| IBIS file ussst2gxxac.ibs created by s2ibis3 verion 1.1
| North Carolina State University, ERL, 2006
| This Model is valid for Commercial Temperature Range 0C<=Tc<=95C
| Valid for DDR2-400/533/667/800/1067 operation
| Part Number   VDD/VDDQ   Package   Architecture
| SCB18T2G160AF   1.8 +0.1/-0.1   84-Ball FBGA   128Meg x 16
| SCB18T2G800AF   1.8 +0.1/-0.1   60-Ball FBGA   256Meg x 8
| SCN18T2G160AF   1.8 +0.1/-0.1   84-Ball FBGA   128Meg x 16
| SCN18T2G800AF   1.8 +0.1/-0.1   60-Ball FBGA   256Meg x 8
| TOPR: Operating Temperature
[IBIS Ver]   3.2
[File name]  ussst2gxxac.ibs
[File Rev]   1.6
[Date]   2016-09-17
[Source]   Simulation of a silicon level SPICE model
[Notes]   IBIS Characteristics for I/O Buffer
   IBIS Model Revision History:
Rev 1.3: 2014-10-14
   - IBIS model file initial creation
Rev 1.3: 2016-09-01
   - update model ODT_75 and ODT_150;
Rev 1.3: 2016-09-05
   - update x16 UDQS#/UDQS/UDM/LDQS#/LDQS/LDM model information;
   - update x8  RDQS#/DM_RDQS model information;
   - add new model RDQS;
Rev 1.4: 2016-09-05
   - correct support speed
   - change RDQS#/DM_RDQS model style
Rev 1.5: 2016-09-08
   - update data to support DDR2-800/1067
Rev 1.6: 2016-09-17
   - split and update "DATA_FULL_800" & "DATA_REDUCED_800"
   and  "DATA_FULL_1067" & "DATA_REDUCED_1067"
   "rising" & "falling" wave data;
   - update ODT "power clamp" data to touch zero current point.
[disclaimer] The IBIS models are for modeling purpose only and are
   subject to change without any notice. UniIC is not
   responsible for any problems the models may cause.
[Copyright]  Copyright 2016 UniIC Semiconductors Corp. All rights reserved
|   Component: SCB18T2G160AF
[Component]   SCB18T2G160AF
[Manufacturer]   UniIC Semiconductors Corp.
| All balls excluding NC, POWER and GND (R[Ohm], L[H], C[F])
[Package]   | FBGA-84 Ball
|Variable   typ   min   max
R_pkg   3.54E-01   2.15E-01   4.22E-01
L_pkg   1.74E-09   9.52E-10   2.26E-09
C_pkg   5.49E-13   3.07E-13   7.49E-13
[Pin]   signal_name model_name   R_pin   L_pin   C_pin
A1   VDD   POWER   NA   NA   NA
A3   VSS   GND   NA   NA   NA
A7   VSSQ   GND   NA   NA   NA
A8   UDQS#   DQ   3.91E-01   1.89E-09   6.31E-13
A9   VDDQ   POWER   NA   NA   NA
B1   DQ14   DQ   3.94E-01   1.93E-09   6.78E-13
B2   VSSQ   GND   NA   NA   NA
B3   UDM   DM   4.00E-01   1.72E-09   6.23E-13
B7   UDQS   DQ   3.85E-01   1.79E-09   6.17E-13
B8   VSSQ   GND   NA   NA   NA
B9   DQ15   DQ   4.04E-01   1.94E-09   6.87E-13
C1   VDDQ   POWER   NA   NA   NA
C2   DQ9   DQ   3.30E-01   1.58E-09   6.19E-13
C3   VDDQ   POWER   NA   NA   NA
C7   VDDQ   POWER   NA   NA   NA
C8   DQ8   DQ   3.86E-01   1.81E-09   6.25E-13
C9   VDDQ   POWER   NA   NA   NA
D1   DQ12   DQ   4.15E-01   2.16E-09   7.19E-13
D2   VSSQ   GND   NA   NA   NA
D3   DQ11   DQ   3.58E-01   1.84E-09   4.33E-13
D7   DQ10   DQ   3.59E-01   1.54E-09   6.33E-13
D8   VSSQ   GND   NA   NA   NA
D9   DQ13   DQ   3.88E-01   1.80E-09   6.09E-13
E1   VDD   POWER   NA   NA   NA
E3   VSS   GND   NA   NA   NA
E7   VSSQ   GND   NA   NA   NA
E8   LDQS#   DQ   3.29E-01   1.47E-09   5.27E-13
E9   VDDQ   POWER   NA   NA   NA
F1   DQ6   DQ   3.57E-01   1.72E-09   6.81E-13
F2   VSSQ   GND   NA   NA   NA
F3   LDM   DM   3.66E-01   1.80E-09   4.94E-13
F7   LDQS   DQ   3.51E-01   1.65E-09   4.51E-13
F8   VSSQ   GND   NA   NA   NA
F9   DQ7   DQ   3.45E-01   1.65E-09   5.83E-13
G1   VDDQ   POWER   NA   NA   NA
G2   DQ1   DQ   3.74E-01   1.80E-09   5.29E-13
G3   VDDQ   POWER   NA   NA   NA
G7   VDDQ   POWER   NA   NA   NA
G8   DQ0   DQ   3.89E-01   1.76E-09   7.05E-13
G9   VDDQ   POWER   NA   NA   NA
H1   DQ4   DQ   4.00E-01   1.95E-09   6.62E-13
H2   VSSQ   GND   NA   NA   NA
H3   DQ3   DQ   3.99E-01   1.92E-09   4.51E-13
H7   DQ2   DQ   3.73E-01   1.57E-09   6.01E-13
H8   VSSQ   GND   NA   NA   NA
H9   DQ5   DQ   3.76E-01   1.57E-09   6.31E-13
J1   VDDL   POWER   NA   NA   NA
J2   VREF   POWER   NA   NA   NA
J3   VSS   GND   NA   NA   NA
J7   VSSDL   GND   NA   NA   NA
J8   CK   CLKCA_RCV   2.92E-01   1.50E-09   4.65E-13
J9   VDD   POWER   NA   NA   NA
K2   CKE   CLKCA_RCV   2.87E-01   1.53E-09   4.36E-13
K3   WE#   CLKCA_RCV   2.26E-01   1.11E-09   3.27E-13
K7   RAS#   CLKCA_RCV   2.27E-01   9.78E-10   3.41E-13
K8   CK#   CLKCA_RCV   2.98E-01   1.41E-09   5.62E-13
K9   ODT   CLKCA_RCV   3.79E-01   1.97E-09   7.49E-13
L1   BA2   CLKCA_RCV   3.69E-01   2.26E-09   5.19E-13
L2   BA0   CLKCA_RCV   3.48E-01   1.83E-09   4.55E-13
L3   BA1   CLKCA_RCV   2.17E-01   9.61E-10   3.07E-13
L7   CAS#   CLKCA_RCV   2.15E-01   9.52E-10   4.00E-13
L8   CS#   CLKCA_RCV   2.95E-01   1.43E-09   5.20E-13
M2   A10   CLKCA_RCV   3.56E-01   1.93E-09   5.14E-13
M3   A1   CLKCA_RCV   3.41E-01   1.90E-09   3.68E-13
M7   A2   CLKCA_RCV   3.40E-01   1.79E-09   4.49E-13
M8   A0   CLKCA_RCV   3.54E-01   1.82E-09   5.67E-13
M9   VDD   POWER   NA   NA   NA
N1   VSS   GND   NA   NA   NA
N2   A3   CLKCA_RCV   3.46E-01   1.82E-09   5.59E-13
N3   A5   CLKCA_RCV   3.56E-01   1.85E-09   5.59E-13
N7   A6   CLKCA_RCV   3.76E-01   1.76E-09   6.49E-13
N8   A4   CLKCA_RCV   3.52E-01   1.90E-09   4.89E-13
P2   A7   CLKCA_RCV   3.86E-01   1.97E-09   6.01E-13
P3   A9   CLKCA_RCV   4.08E-01   2.11E-09   4.37E-13
P7   A11   CLKCA_RCV   4.01E-01   2.17E-09   5.49E-13
P8   A8   CLKCA_RCV   3.87E-01   1.85E-09   5.76E-13
P9   VSS   GND   NA   NA   NA
R1   VDD   POWER   NA   NA   NA
R2   A12   CLKCA_RCV   4.22E-01   2.07E-09   6.47E-13
R8   A13   CLKCA_RCV   3.99E-01   1.97E-09   5.55E-13
|*****************************  Diff Pin  *************************************
[Diff Pin]  inv_pin  vdiff   tdelay_typ  tdelay_min  tdelay_max
J8   K8   0.2500V   NA   NA   NA
B7   A8   0.2500V   NA   NA   NA
F7   E8   0.2500V   NA   NA   NA
|  Pins B7 and A8 are a differential I/O only when DQS# is enabled via MRS
|  If DQS# is disabled, then B7(UDQS) is a single ended I/O and A8 is a NC
|  Pins F7 and E8 are a differential I/O only when DQS# is enabled via MRS
|  If DQS# is disabled, then F7(LDQS) is a single ended I/O and E8 is a NC
|   Component SCB18T2G800AF
[Component]   SCB18T2G800AF
[Manufacturer]   UniIC Semiconductors Corp.
[Package]   | FBGA-60 Ball
|Variable   typ   min   max
R_pkg   4.44E-01   3.39E-01   5.16E-01
L_pkg   1.80E-09   1.34E-09   2.17E-09
C_pkg   5.78E-13   2.96E-13   8.56E-13
[Pin]   signal_name model_name   R_pin   L_pin   C_pin
A1   VDD   POWER   NA   NA   NA
A2   RDQS#   RDQS#   4.96E-01   1.97E-09   6.07E-13
A3   VSS   GND   NA   NA   NA
A7   VSSQ   GND   NA   NA   NA
A8   DQS#   DQ   4.73E-01   1.84E-09   6.59E-13
A9   VDDQ   POWER   NA   NA   NA
B1   DQ6   DQ   4.92E-01   1.88E-09   7.44E-13
B2   VSSQ   GND   NA   NA   NA
B3   DM_RDQS   DM_RDQS   4.94E-01   1.87E-09   5.97E-13
B7   DQS   DQ   4.79E-01   1.80E-09   6.15E-13
B8   VSSQ   GND   NA   NA   NA
B9   DQ7   DQ   4.95E-01   1.95E-09   8.56E-13
C1   VDDQ   POWER   NA   NA   NA
C2   DQ1   DQ   4.80E-01   1.91E-09   6.59E-13
C3   VDDQ   POWER   NA   NA   NA
C7   VDDQ   POWER   NA   NA   NA
C8   DQ0   DQ   4.92E-01   1.87E-09   6.13E-13
C9   VDDQ   POWER   NA   NA   NA
D1   DQ4   DQ   5.16E-01   1.92E-09   7.50E-13
D2   VSSQ   GND   NA   NA   NA
D3   DQ3   DQ   4.76E-01   1.71E-09   7.34E-13
D7   DQ2   DQ   4.69E-01   1.69E-09   7.66E-13
D8   VSSQ   GND   NA   NA   NA
D9   DQ5   DQ   5.14E-01   1.92E-09   7.82E-13
E1   VDDL   POWER   NA   NA   NA
E2   VREF   POWER   NA   NA   NA
E3   VSS   GND   NA   NA   NA
E7   VSSDL   GND   NA   NA   NA
E8   CK   CLKCA_RCV   4.09E-01   1.68E-09   6.82E-13
E9   VDD   POWER   NA   NA   NA
F2   CKE   CLKCA_RCV   4.33E-01   1.91E-09   6.25E-13
F3   WE#   CLKCA_RCV   4.06E-01   1.83E-09   5.01E-13
F7   RAS#   CLKCA_RCV   3.39E-01   1.34E-09   2.96E-13
F8   CK#   CLKCA_RCV   4.12E-01   1.69E-09   6.27E-13
F9   ODT   CLKCA_RCV   4.59E-01   2.13E-09   7.14E-13
G1   BA2   CLKCA_RCV   4.69E-01   2.17E-09   7.10E-13
G2   BA0   CLKCA_RCV   4.17E-01   1.75E-09   5.68E-13
G3   BA1   CLKCA_RCV   4.39E-01   1.69E-09   6.38E-13
G7   CAS#   CLKCA_RCV   3.91E-01   1.42E-09   4.04E-13
G8   CS#   CLKCA_RCV   4.28E-01   1.74E-09   5.05E-13
H2   A10   CLKCA_RCV   4.43E-01   1.81E-09   5.46E-13
H3   A1   CLKCA_RCV   4.28E-01   1.94E-09   3.78E-13
H7   A2   CLKCA_RCV   4.12E-01   1.79E-09   4.44E-13
H8   A0   CLKCA_RCV   4.53E-01   1.80E-09   6.26E-13
H9   VDD   POWER   NA   NA   NA
J1   VSS   GND   NA   NA   NA
J2   A3   CLKCA_RCV   4.35E-01   1.79E-09   5.23E-13
J3   A5   CLKCA_RCV   3.52E-01   1.38E-09   3.72E-13
J7   A6   CLKCA_RCV   4.08E-01   1.76E-09   4.50E-13
J8   A4   CLKCA_RCV   4.49E-01   1.91E-09   5.16E-13
K2   A7   CLKCA_RCV   4.48E-01   1.74E-09   6.39E-13
K3   A9   CLKCA_RCV   4.07E-01   1.75E-09   4.69E-13
K7   A11   CLKCA_RCV   4.26E-01   1.96E-09   4.05E-13
K8   A8   CLKCA_RCV   4.34E-01   1.62E-09   5.18E-13
K9   VSS   GND   NA   NA   NA
L1   VDD   POWER   NA   NA   NA
L2   A12   CLKCA_RCV   4.16E-01   1.82E-09   4.13E-13
L3   A14   CLKCA_RCV   4.51E-01   1.98E-09   5.04E-13
L8   A13   CLKCA_RCV   4.15E-01   1.66E-09   5.04E-13
|*****************************  Diff Pin  *************************************
[Diff Pin]  inv_pin  vdiff   tdelay_typ  tdelay_min  tdelay_max
E8   F8   0.2500V   NA   NA   NA
B7   A8   0.2500V   NA   NA   NA
|  Pins B7 and A8 are a differential I/O only when DQS# is enabled via MRS
|  If DQS# is disabled, then B7 (DQS) is a single ended I/O and A8 is a NC
|B3   A2   0.2500V   NA   NA   NA
|  Pins B3 and A2 (RDQS,RDQS#) are a differential output only if RDQS and
|  Differential Strobe MRS options are enabled
|  If RDQS is disabled, then B3 (DM) is single input with ODT and A2 is a NC
|   Component: SCN18T2G160AF
[Component]   SCN18T2G160AF
[Manufacturer]   UniIC Semiconductors Corp.
| All balls excluding NC, POWER and GND (R[Ohm], L[H], C[F])
[Package]   | FBGA-84 Ball
|Variable   typ   min   max
R_pkg   3.54E-01   2.15E-01   4.22E-01
L_pkg   1.74E-09   9.52E-10   2.26E-09
C_pkg   5.49E-13   3.07E-13   7.49E-13
[Pin]   signal_name model_name   R_pin   L_pin   C_pin
A1   VDD   POWER   NA   NA   NA
A3   VSS   GND   NA   NA   NA
A7   VSSQ   GND   NA   NA   NA
A8   UDQS#   DQ   3.91E-01   1.89E-09   6.31E-13
A9   VDDQ   POWER   NA   NA   NA
B1   DQ14   DQ   3.94E-01   1.93E-09   6.78E-13
B2   VSSQ   GND   NA   NA   NA
B3   UDM   DM   4.00E-01   1.72E-09   6.23E-13
B7   UDQS   DQ   3.85E-01   1.79E-09   6.17E-13
B8   VSSQ   GND   NA   NA   NA
B9   DQ15   DQ   4.04E-01   1.94E-09   6.87E-13
C1   VDDQ   POWER   NA   NA   NA
C2   DQ9   DQ   3.30E-01   1.58E-09   6.19E-13
C3   VDDQ   POWER   NA   NA   NA
C7   VDDQ   POWER   NA   NA   NA
C8   DQ8   DQ   3.86E-01   1.81E-09   6.25E-13
C9   VDDQ   POWER   NA   NA   NA
D1   DQ12   DQ   4.15E-01   2.16E-09   7.19E-13
D2   VSSQ   GND   NA   NA   NA
D3   DQ11   DQ   3.58E-01   1.84E-09   4.33E-13
D7   DQ10   DQ   3.59E-01   1.54E-09   6.33E-13
D8   VSSQ   GND   NA   NA   NA
D9   DQ13   DQ   3.88E-01   1.80E-09   6.09E-13
E1   VDD   POWER   NA   NA   NA
E3   VSS   GND   NA   NA   NA
E7   VSSQ   GND   NA   NA   NA
E8   LDQS#   DQ   3.29E-01   1.47E-09   5.27E-13
E9   VDDQ   POWER   NA   NA   NA
F1   DQ6   DQ   3.57E-01   1.72E-09   6.81E-13
F2   VSSQ   GND   NA   NA   NA
F3   LDM   DM   3.66E-01   1.80E-09   4.94E-13
F7   LDQS   DQ   3.51E-01   1.65E-09   4.51E-13
F8   VSSQ   GND   NA   NA   NA
F9   DQ7   DQ   3.45E-01   1.65E-09   5.83E-13
G1   VDDQ   POWER   NA   NA   NA
G2   DQ1   DQ   3.74E-01   1.80E-09   5.29E-13
G3   VDDQ   POWER   NA   NA   NA
G7   VDDQ   POWER   NA   NA   NA
G8   DQ0   DQ   3.89E-01   1.76E-09   7.05E-13
G9   VDDQ   POWER   NA   NA   NA
H1   DQ4   DQ   4.00E-01   1.95E-09   6.62E-13
H2   VSSQ   GND   NA   NA   NA
H3   DQ3   DQ   3.99E-01   1.92E-09   4.51E-13
H7   DQ2   DQ   3.73E-01   1.57E-09   6.01E-13
H8   VSSQ   GND   NA   NA   NA
H9   DQ5   DQ   3.76E-01   1.57E-09   6.31E-13
J1   VDDL   POWER   NA   NA   NA
J2   VREF   POWER   NA   NA   NA
J3   VSS   GND   NA   NA   NA
J7   VSSDL   GND   NA   NA   NA
J8   CK   CLKCA_RCV   2.92E-01   1.50E-09   4.65E-13
J9   VDD   POWER   NA   NA   NA
K2   CKE   CLKCA_RCV   2.87E-01   1.53E-09   4.36E-13
K3   WE#   CLKCA_RCV   2.26E-01   1.11E-09   3.27E-13
K7   RAS#   CLKCA_RCV   2.27E-01   9.78E-10   3.41E-13
K8   CK#   CLKCA_RCV   2.98E-01   1.41E-09   5.62E-13
K9   ODT   CLKCA_RCV   3.79E-01   1.97E-09   7.49E-13
L1   BA2   CLKCA_RCV   3.69E-01   2.26E-09   5.19E-13
L2   BA0   CLKCA_RCV   3.48E-01   1.83E-09   4.55E-13
L3   BA1   CLKCA_RCV   2.17E-01   9.61E-10   3.07E-13
L7   CAS#   CLKCA_RCV   2.15E-01   9.52E-10   4.00E-13
L8   CS#   CLKCA_RCV   2.95E-01   1.43E-09   5.20E-13
M2   A10   CLKCA_RCV   3.56E-01   1.93E-09   5.14E-13
M3   A1   CLKCA_RCV   3.41E-01   1.90E-09   3.68E-13
M7   A2   CLKCA_RCV   3.40E-01   1.79E-09   4.49E-13
M8   A0   CLKCA_RCV   3.54E-01   1.82E-09   5.67E-13
M9   VDD   POWER   NA   NA   NA
N1   VSS   GND   NA   NA   NA
N2   A3   CLKCA_RCV   3.46E-01   1.82E-09   5.59E-13
N3   A5   CLKCA_RCV   3.56E-01   1.85E-09   5.59E-13
N7   A6   CLKCA_RCV   3.76E-01   1.76E-09   6.49E-13
N8   A4   CLKCA_RCV   3.52E-01   1.90E-09   4.89E-13
P2   A7   CLKCA_RCV   3.86E-01   1.97E-09   6.01E-13
P3   A9   CLKCA_RCV   4.08E-01   2.11E-09   4.37E-13
P7   A11   CLKCA_RCV   4.01E-01   2.17E-09   5.49E-13
P8   A8   CLKCA_RCV   3.87E-01   1.85E-09   5.76E-13
P9   VSS   GND   NA   NA   NA
R1   VDD   POWER   NA   NA   NA
R2   A12   CLKCA_RCV   4.22E-01   2.07E-09   6.47E-13
R8   A13   CLKCA_RCV   3.99E-01   1.97E-09   5.55E-13
|*****************************  Diff Pin  *************************************
[Diff Pin]  inv_pin  vdiff   tdelay_typ  tdelay_min  tdelay_max
J8   K8   0.2500V   NA   NA   NA
B7   A8   0.2500V   NA   NA   NA
F7   E8   0.2500V   NA   NA   NA
|  Pins B7 and A8 are a differential I/O only when DQS# is enabled via MRS
|  If DQS# is disabled, then B7(UDQS) is a single ended I/O and A8 is a NC
|  Pins F7 and E8 are a differential I/O only when DQS# is enabled via MRS
|  If DQS# is disabled, then F7(LDQS) is a single ended I/O and E8 is a NC
|   Component SCN18T2G800AF
[Component]   SCN18T2G800AF
[Manufacturer]   UniIC Semiconductors Corp.
[Package]   | FBGA-60 Ball
|Variable   typ   min   max
R_pkg   4.44E-01   3.39E-01   5.16E-01
L_pkg   1.80E-09   1.34E-09   2.17E-09
C_pkg   5.78E-13   2.96E-13   8.56E-13
[Pin]   signal_name model_name   R_pin   L_pin   C_pin
A1   VDD   POWER   NA   NA   NA
A2   RDQS#   RDQS#   4.96E-01   1.97E-09   6.07E-13
A3   VSS   GND   NA   NA   NA
A7   VSSQ   GND   NA   NA   NA
A8   DQS#   DQ   4.73E-01   1.84E-09   6.59E-13
A9   VDDQ   POWER   NA   NA   NA
B1   DQ6   DQ   4.92E-01   1.88E-09   7.44E-13
B2   VSSQ   GND   NA   NA   NA
B3   DM_RDQS   DM_RDQS   4.94E-01   1.87E-09   5.97E-13
B7   DQS   DQ   4.79E-01   1.80E-09   6.15E-13
B8   VSSQ   GND   NA   NA   NA
B9   DQ7   DQ   4.95E-01   1.95E-09   8.56E-13
C1   VDDQ   POWER   NA   NA   NA
C2   DQ1   DQ   4.80E-01   1.91E-09   6.59E-13
C3   VDDQ   POWER   NA   NA   NA
C7   VDDQ   POWER   NA   NA   NA
C8   DQ0   DQ   4.92E-01   1.87E-09   6.13E-13
C9   VDDQ   POWER   NA   NA   NA
D1   DQ4   DQ   5.16E-01   1.92E-09   7.50E-13
D2   VSSQ   GND   NA   NA   NA
D3   DQ3   DQ   4.76E-01   1.71E-09   7.34E-13
D7   DQ2   DQ   4.69E-01   1.69E-09   7.66E-13
D8   VSSQ   GND   NA   NA   NA
D9   DQ5   DQ   5.14E-01   1.92E-09   7.82E-13
E1   VDDL   POWER   NA   NA   NA
E2   VREF   POWER   NA   NA   NA
E3   VSS   GND   NA   NA   NA
E7   VSSDL   GND   NA   NA   NA
E8   CK   CLKCA_RCV   4.09E-01   1.68E-09   6.82E-13
E9   VDD   POWER   NA   NA   NA
F2   CKE   CLKCA_RCV   4.33E-01   1.91E-09   6.25E-13
F3   WE#   CLKCA_RCV   4.06E-01   1.83E-09   5.01E-13
F7   RAS#   CLKCA_RCV   3.39E-01   1.34E-09   2.96E-13
F8   CK#   CLKCA_RCV   4.12E-01   1.69E-09   6.27E-13
F9   ODT   CLKCA_RCV   4.59E-01   2.13E-09   7.14E-13
G1   BA2   CLKCA_RCV   4.69E-01   2.17E-09   7.10E-13
G2   BA0   CLKCA_RCV   4.17E-01   1.75E-09   5.68E-13
G3   BA1   CLKCA_RCV   4.39E-01   1.69E-09   6.38E-13
G7   CAS#   CLKCA_RCV   3.91E-01   1.42E-09   4.04E-13
G8   CS#   CLKCA_RCV   4.28E-01   1.74E-09   5.05E-13
H2   A10   CLKCA_RCV   4.43E-01   1.81E-09   5.46E-13
H3   A1   CLKCA_RCV   4.28E-01   1.94E-09   3.78E-13
H7   A2   CLKCA_RCV   4.12E-01   1.79E-09   4.44E-13
H8   A0   CLKCA_RCV   4.53E-01   1.80E-09   6.26E-13
H9   VDD   POWER   NA   NA   NA
J1   VSS   GND   NA   NA   NA
J2   A3   CLKCA_RCV   4.35E-01   1.79E-09   5.23E-13
J3   A5   CLKCA_RCV   3.52E-01   1.38E-09   3.72E-13
J7   A6   CLKCA_RCV   4.08E-01   1.76E-09   4.50E-13
J8   A4   CLKCA_RCV   4.49E-01   1.91E-09   5.16E-13
K2   A7   CLKCA_RCV   4.48E-01   1.74E-09   6.39E-13
K3   A9   CLKCA_RCV   4.07E-01   1.75E-09   4.69E-13
K7   A11   CLKCA_RCV   4.26E-01   1.96E-09   4.05E-13
K8   A8   CLKCA_RCV   4.34E-01   1.62E-09   5.18E-13
K9   VSS   GND   NA   NA   NA
L1   VDD   POWER   NA   NA   NA
L2   A12   CLKCA_RCV   4.16E-01   1.82E-09   4.13E-13
L3   A14   CLKCA_RCV   4.51E-01   1.98E-09   5.04E-13
L8   A13   CLKCA_RCV   4.15E-01   1.66E-09   5.04E-13
|*****************************  Diff Pin  *************************************
[Diff Pin]  inv_pin  vdiff   tdelay_typ  tdelay_min  tdelay_max
E8   F8   0.2500V   NA   NA   NA
B7   A8   0.2500V   NA   NA   NA
|  Pins B7 and A8 are a differential I/O only when DQS# is enabled via MRS
|  If DQS# is disabled, then B7 (DQS) is a single ended I/O and A8 is a NC
|B3   A2   0.2500V   NA   NA   NA
|  Pins B3 and A2 (RDQS,RDQS#) are a differential output only if RDQS and
|  Differential Strobe MRS options are enabled
|  If RDQS is disabled, then B3 (DM) is single input with ODT and A2 is a NC
|*****************************  Model Selector ********************************
[Model Selector]   DQ
DATA_FULL_800   Full-Strength Output Driver (ODT Off)(400/533/667/800 Mbps)
DATA_REDUCED_800   60%-Strength Output Driver (ODT Off)(400/533/667/800 Mbps)
DATA_FULL_1067   Full-Strength Output Driver (ODT Off)(1067 Mbps)
DATA_REDUCED_1067   60%-Strength Output Driver (ODT Off)(1067 Mbps)
DATA_RCV   Data/Data Strobe/Data Mask Receiver
ODT_50   ODT 50 Ohm
ODT_75   ODT 75 Ohm
ODT_150   ODT 150 Ohm
[Model Selector]   DM
DATA_RCV   Data/Data Strobe/Data Mask Receiver
ODT_50   ODT 50 Ohm
ODT_75   ODT 75 Ohm
ODT_150   ODT 150 Ohm
[Model Selector]   RDQS#
NC_DQ   Not Used if either RDQS or Diff. Strobe are disabled
DATA_FULL_800   Full-Strength Output Driver (ODT Off)(400/533/667/800 Mbps)
DATA_REDUCED_800   60%-Strength Output Driver (ODT Off)(400/533/667/800 Mbps)
DATA_FULL_1067   Full-Strength Output Driver (ODT Off)(1067 Mbps)
DATA_REDUCED_1067   60%-Strength Output Driver (ODT Off)(1067 Mbps)
|If RDQS is enabled, then RDQS# is OUTPUT only (DATA_FULL and DATA_REDUCED)
|If RDQS is disabled, then RDQS# is a NC
[Model Selector]   DM_RDQS
DATA_FULL_800   Full-Strength Output Driver (ODT Off)(400/533/667/800 Mbps)
DATA_REDUCED_800   60%-Strength Output Driver (ODT Off)(400/533/667/800 Mbps)
DATA_FULL_1067   Full-Strength Output Driver (ODT Off)(1067 Mbps)
DATA_REDUCED_1067   60%-Strength Output Driver (ODT Off)(1067 Mbps)
DATA_RCV   Data/Data Strobe/Data Mask Receiver
ODT_50   ODT 50 Ohm
ODT_75   ODT 75 Ohm
ODT_150   ODT 150 Ohm
| Models and submodels in the file (10): DATA_FULL_800 (I/O), DATA_REDUCED_800 (I/O), DATA_FULL_1067 (I/O), DATA_REDUCED_1067 (I/O), DATA_RCV (Input), NC_DQ (Input), ODT_150 (Input), ODT_75 (Input), ODT_50 (Input), CLKCA_RCV (Input)
